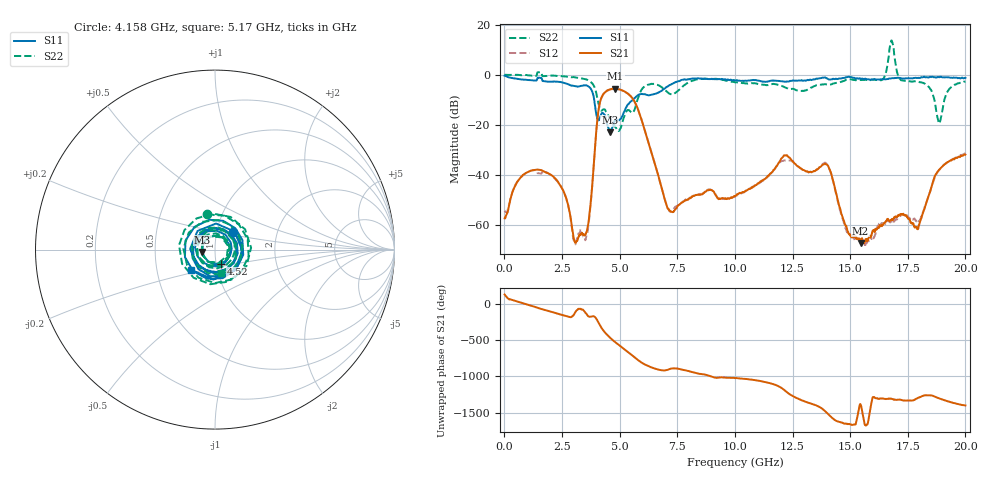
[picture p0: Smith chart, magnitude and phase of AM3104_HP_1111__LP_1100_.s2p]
!Created with skrf (http://scikit-rf.org).
# Hz S RI R 50.0
!freq ReS11 ImS11 ReS21 ImS21 ReS12 ImS12 ReS22 ImS22
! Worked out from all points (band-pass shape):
!   1601 points, 10 MHz to 20 GHz, reference 50 ohm
!   highest |S21| = -5.61 dB at 4.808 GHz (marker M1); lowest = -67.2 dB at 15.45 GHz (marker M2)
!   |S21| within 3 dB of the highest: 4.242 GHz to 5.48 GHz (1.237 GHz wide, 25.5 % of centre)
!   lowest |S11| = -23.0 dB at 4.57 GHz (marker M3), VSWR 1.15, Z = 43.5 - j1.15 ohm
!   |S11| at or under -10 dB: 3.896 GHz to 5.577 GHz (1.681 GHz wide, 35.5 % of centre)
!   |S22| runs from -22.5 to 13.6 dB; largest |S21 - S12| = 0.055
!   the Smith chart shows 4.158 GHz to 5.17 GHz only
!   S11 on the Smith chart (normalised r, x): 4.158 GHz: 1.20, +0.24; 4.52 GHz: 1.05, -0.17; 5.17 GHz: 0.75, -0.17
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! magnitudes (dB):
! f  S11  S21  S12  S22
! 10 MHz  -0.4  -57.4  -54.5  -0.1
! 634.7 MHz  -1.8  -41.9  -41.9  -0.1
! 1.547 GHz  -1.3  -38.0  -39.5  0.9
! 3.346 GHz  -4.5  -63.4  -63.7  -1.5
! 3.633 GHz  -4.6  -59.9  -61.0  -2.3
! 4.158 GHz  -16.9  -10.7  -10.7  -14.0
! 4.52 GHz  -21.4  -6.1  -6.2  -16.4
! 4.57 GHz  -23.0  -5.9  -6.1  -17.5
! 4.808 GHz  -18.5  -5.6  -5.7  -20.9
! 5.17 GHz  -15.2  -6.5  -6.5  -17.4
! 6.682 GHz  -7.2  -40.5  -40.5  -4.2
! 7.256 GHz  -3.8  -54.8  -54.1  -8.0
! 10.01 GHz  -2.4  -48.6  -48.7  -3.1
! 12.17 GHz  -2.8  -32.3  -34.2  -5.1
! 13.34 GHz  -2.1  -38.9  -38.9  -5.1
! 14.03 GHz  -1.7  -36.3  -36.2  -4.0
! 14.83 GHz  -1.0  -60.5  -62.2  -2.1
! 15.45 GHz  -1.6  -67.2  -64.0  -2.2
! 16.68 GHz  -1.6  -58.2  -58.6  7.3
! 17.93 GHz  -1.3  -61.6  -58.3  -2.7
! 18.86 GHz  -1.0  -38.0  -38.1  -19.5
! 20 GHz  -1.3  -31.9  -31.5  -2.7
